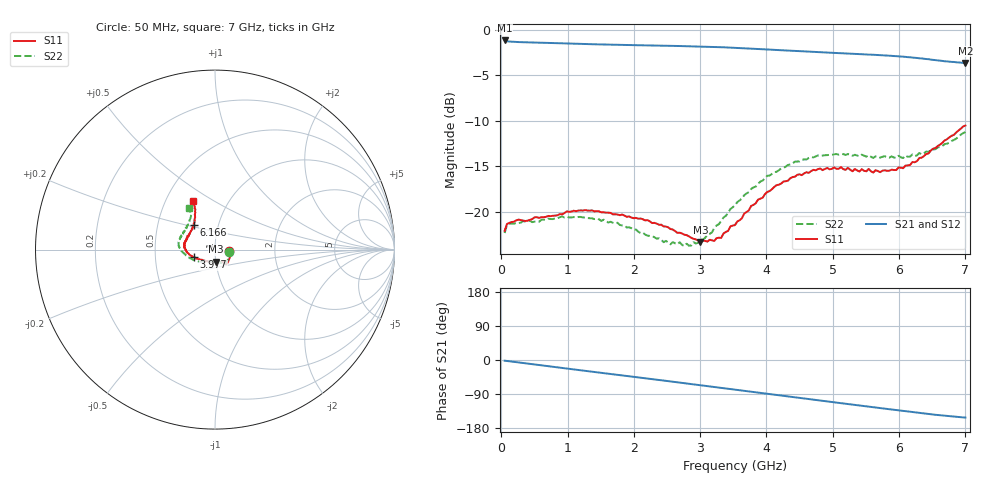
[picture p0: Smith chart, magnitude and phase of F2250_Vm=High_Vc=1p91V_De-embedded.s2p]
! Integrated Device Technology
! Corporate Headquarters
! 6024 Silver Creek Valley Road
! San Jose, CA 95138  USA
! Phone:  1-408-284-8200
! Toll Free:  1-800-223-1366
! Webpage:  http://www.idt.com/
! Timing and RF Division
! 515 Groton Road, Suite 102
! Westford, MA 01886-6024
! Device:  F2250
! Description: Voltage Variable RF Attenuator
! Frequency:  50.0 -  6000.00 MHz
! Package:  3x3 mm Thin QFN Plastic Package: 16 pin
! Ports:  2 RF, 3 DC
!  Pin  1  = GND
!  Pin  2  = NC
!  Pin  3  = RF1  = Port 1
!  Pin  4  = NC
!  Pin  5  = GND
!  Pin  6  = GND
!  Pin  7  = GND
!  Pin  8  = GND
!  Pin  9  = NC
!  Pin 10  = RF2  = Port 2
!  Pin 11  = NC
!  Pin 12  = GND
!  Pin 13  = GND
!  Pin 14  = VCNTRL
!  Pin 15  = VDD
!  Pin 16  = VMODE
! Vcntrl:  1.910 Volts
! Vmode:  +3.300 Volts
! Vdd:  +3.30  Volts
! Current:  1.321 mA
! Data:  The device was measured on a the F2250 evaluation board which has
!  individual transmission lines to the RF pins.  Data was collected
!  using a calibrated network analyzer.  The evaluation board was
!  de-embedded using a TRL calibration technique.
!  The reference plane is the edge of the package pin.
! Misc:  SN 10
!  Action Tracker AT0258
! Date Measured:  2014-11-26
! Date:  2015-10-15  MJV
! Note:
!  Integrated Device Technology supplies this data as a sample of measured
!  data at the package pin for this product.  Your particular data for this
!  product may vary.
!  Data was taken at 25 degrees C.
!  Integrated Device Technology reserves the right to change this data at anytime.
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# GHz S dB R 50
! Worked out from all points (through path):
!   201 points, 50 MHz to 7 GHz, reference 50 ohm
!   highest |S21| = -1.15 dB at 50 MHz (marker M1); lowest = -3.6 dB at 7 GHz (marker M2)
!   group delay of S21, straight-line fit = 61.1 ps
!   lowest |S11| = -23.3 dB at 3.004 GHz (marker M3), VSWR 1.15, Z = 50.1 - j6.84 ohm
!   |S11| at or under -10 dB: start of sweep to end of sweep
!   |S22| runs from -23.8 to -11.2 dB; largest |S21 - S12| = 0.0019
!   S11 on the Smith chart (normalised r, x): 50 MHz: 1.17, -0.02; 3.977 GHz: 0.79, -0.07; 6.166 GHz: 0.76, +0.22; 7 GHz: 0.68, +0.41
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0.05  -22.11 -7.2  -1.15 -1.8  -1.15 -1.8  -22.35 -8.1
0.08475  -21.36 -6.8  -1.23 -2.5  -1.23 -2.5  -21.50 -7.4
0.1195  -21.23 -7.4  -1.27 -3.3  -1.27 -3.3  -21.32 -7.3
0.6755  -20.56 -29.6  -1.41 -15.7  -1.41 -15.7  -20.91 -32.3
1.2315  -19.87 -47.4  -1.53 -27.9  -1.53 -27.9  -20.63 -54.9
1.75275  -20.31 -54.3  -1.63 -39.1  -1.63 -39.1  -21.22 -64.0
2.37825  -21.43 -56.2  -1.71 -52.7  -1.72 -52.7  -22.92 -71.0
2.691  -22.31 -65.6  -1.76 -59.6  -1.76 -59.6  -23.36 -83.9
2.7605  -22.53 -67.3  -1.77 -61.2  -1.77 -61.2  -23.79 -87.8
3.00375  -23.33 -85.0  -1.81 -66.6  -1.81 -66.7  -23.06 -106.9
3.1775  -23.15 -98.5  -1.85 -70.6  -1.85 -70.6  -22.28 -120.5
3.3165  -22.88 -115.5  -1.89 -73.7  -1.88 -73.8  -21.02 -130.7
3.4555  -21.62 -128.7  -1.93 -76.9  -1.93 -76.9  -19.71 -139.2
3.525  -21.47 -133.4  -1.95 -78.4  -1.95 -78.5  -19.29 -142.7
3.97675  -18.07 -160.5  -2.12 -88.6  -2.12 -88.7  -16.31 -163.5
4.4285  -16.14 -174.7  -2.30 -98.6  -2.31 -98.6  -14.49 -177.8
4.7065  -15.39 177.6  -2.40 -104.7  -2.40 -104.7  -14.02 176.0
5.054  -15.27 169.1  -2.53 -112.4  -2.53 -112.4  -13.65 168.4
5.85325  -15.48 142.3  -2.83 -129.9  -2.83 -130.0  -14.05 149.1
6.166  -14.85 130.5  -3.00 -136.8  -3.00 -136.8  -13.93 140.5
6.54825  -12.98 120.2  -3.30 -144.6  -3.30 -144.7  -13.12 128.3
7  -10.52 114.4  -3.63 -152.0  -3.64 -152.1  -11.23 121.7
